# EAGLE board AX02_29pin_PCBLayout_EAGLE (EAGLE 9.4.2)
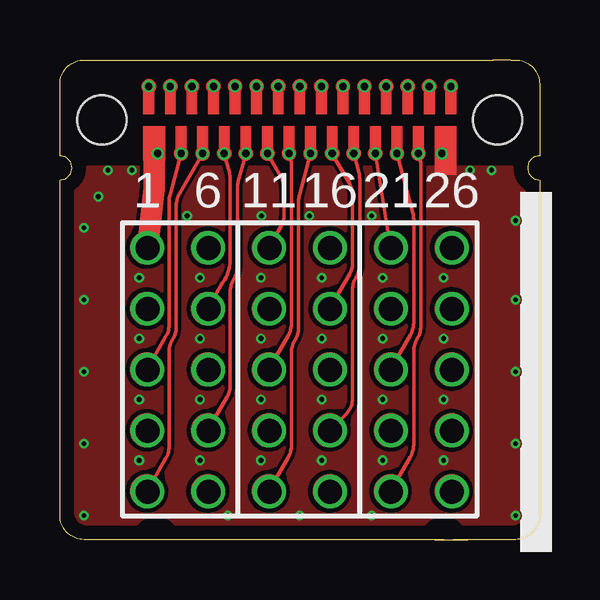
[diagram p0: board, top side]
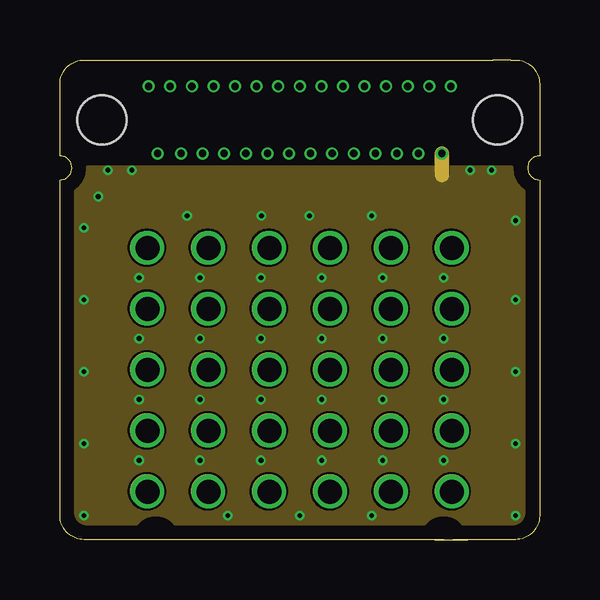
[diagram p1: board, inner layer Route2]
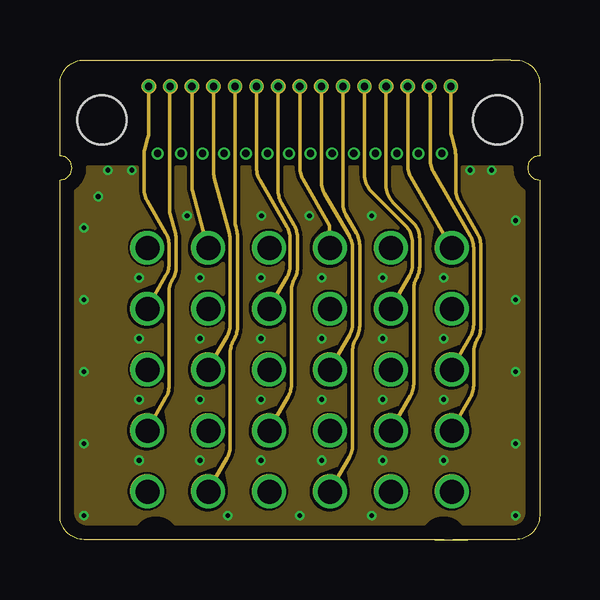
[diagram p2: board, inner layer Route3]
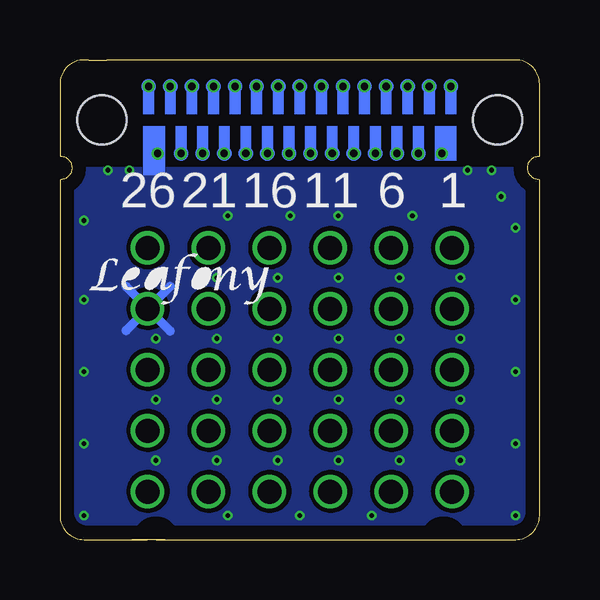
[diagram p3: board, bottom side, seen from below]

Size 20 x 20 mm. Coordinates in mm from the lower left corner, seen from the top.
Outline: 6,20 1,20 arc90 0,19 0,16 arc-180 0,15 0,1 arc90 1,0 16,0
Outline: 5.7,20 16,20
Outline: 15.05,20 18.05,20 18.8,20 19,20 arc-90 20,19 20,16 arc180 20,15 20,1 arc-90 19,0 16.38,0
Outline: 15.62,0 17,0
Copper layers (1*2+3*16): Top 0.035mm / dielectric 0.15mm / Route2 0.035mm / dielectric 0.15mm / Route3 0.035mm / dielectric 0.2mm / Bottom 0.035mm
Design rules "default *": minimum track width 0.01mm, minimum drill 0.01mm, track to track 0.01mm, track to pad 0.01mm, pad to pad 0.01mm, via to via 0.01mm, smd to smd 0.01mm, copper to edge 0.01mm, drill to drill 0.01mm, minimum pad ring 0.1mm, minimum via ring 0.1mm, stop-mask expansion 4mil, vias tented up to drill 0mil, thermal gap 10mil
Net classes: 0 default: width 0.15 mm, drill 0.3 mm; 1 power: width 0.15 mm, drill 0.3 mm

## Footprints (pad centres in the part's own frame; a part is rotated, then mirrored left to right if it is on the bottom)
29PAD = drill 0.3 pad 0.3: 3.3V -5.925,-1.4; A0 -4.5,1.4; A1 -3.6,1.4; A2 -2.7,1.4; A3 -1.8,1.4; A4 -0.9,1.4; A5 0,1.4; AREF -5.4,1.4; D0 0.9,1.4; D1 1.8,1.4; D2 2.7,1.4; D3 3.6,1.4; D4 4.5,1.4; D5 5.4,1.4; D6 -3.15,-1.4; D7 -2.25,-1.4; D8 -1.35,-1.4; D9 -0.45,-1.4; D10 0.45,-1.4; D11 1.35,-1.4; D12 2.25,-1.4; D13 3.15,-1.4; GRD 5.925,-1.4; RESET -4.05,-1.4; SDA 4.05,-1.4; SDL 4.95,-1.4; SWCLK 6.3,1.4; SWDIO -6.3,1.4; VBUS -4.95,-1.4 | hole 2.05: -8.25,0; 8.25,0
30PAD = drill 1 pad 1.4: 3.3V -6.35,12.16; 30PAD 6.35,2; A0 -3.81,12.16; A1 -3.81,7.08; A2 -3.81,2; A3 -1.27,9.62; A4 -1.27,4.54; A5 1.27,12.16; AREF -6.35,4.54; D0 1.27,7.08; D1 1.27,2; D2 3.81,9.62; D3 3.81,4.54; D4 6.35,12.16; D5 6.35,7.08; D6 -3.81,9.62; D7 -3.81,4.54; D8 -1.27,12.16; D9 -1.27,7.08; D10 -1.27,2; D11 1.27,9.62; D12 1.27,4.54; D13 3.81,12.16; GRD 6.35,9.62; REST -6.35,2; SDA 3.81,7.08; SDL 3.81,2; SWCLK 6.35,4.54; SWDIO -6.35,9.62; VBUS -6.35,7.08

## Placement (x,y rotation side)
E$1  [29PAD]  10,17.5 0 top
E$2  [30PAD]  10,0 0 top

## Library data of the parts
E$1 E$2 = 29PAD

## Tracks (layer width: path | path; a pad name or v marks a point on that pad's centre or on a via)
3.3V
  Top 0.9: 3.65,12.16 3.92,14.64 arc7 3.92,14.76 3.92,16.52
A0
  Route3 0.15: 6.17,12.17 5.53,14.53 arc-15 5.5,14.79 5.5,18.9
A1
  Route3 0.15: 6.4,18.9 6.4,15.36 arc15 6.43,15.1 7.07,12.74 arc-15 7.1,12.48 7.1,8.98 arc-30 6.97,8.48 6.17,7.09
A2
  Route3 0.15: 7.3,18.9 7.3,13.28 arc15 7.33,13.02 7.37,12.9 arc-15 7.4,12.64 7.4,8.85 arc-30 7.27,8.35 7.23,8.29 arc30 7.1,7.79 7.1,3.9 arc-30 6.97,3.4 6.17,2.01
A3
  Route3 0.15: 8.71,9.63 9.47,10.95 arc30 9.6,11.45 9.6,12.53 arc30 9.47,13.03 8.33,14.99 arc-30 8.2,15.49 8.2,18.9
A4
  Route3 0.15: 9.1,18.9 9.1,14.54 arc30 9.23,14.04 9.77,13.12 arc-30 9.9,12.62 9.9,11.32 arc-30 9.78,10.86 | 9.78,10.86 | 9.78,10.86 arc30 9.65,10.39 9.65,6.46 arc-30 9.52,5.96 8.71,4.55
A5
  Route3 0.15: 11.25,12.17 11.25,13.1 10.13,15.03 arc-30 10,15.53 10,18.9
AREF
  Route3 0.15: 3.63,4.55 4.42,5.92 arc30 4.55,6.42 4.55,10.32 arc-30 4.68,10.82 4.72,10.88 arc30 4.85,11.38 4.85,12.49 arc15 4.82,12.75 4.6,13.57 arc-15 4.56,13.83 4.56,18.49 arc-5 4.56,18.51 4.6,18.9
D0
  Route3 0.15: 11.25,7.09 12.07,8.51 arc30 12.2,9.01 12.2,12.15 arc30 12.07,12.65 11.03,14.44 arc-30 10.9,14.94 10.9,18.9
D1
  Route3 0.15: 11.25,2.01 12.07,3.43 arc30 12.2,3.93 12.2,7.86 arc-30 12.33,8.36 12.37,8.41 arc30 12.5,8.91 12.5,12.28 arc30 12.37,12.78 11.93,13.52 arc-30 11.8,14.02 11.8,18.9
D2
  Route3 0.15: 13.79,9.63 14.57,10.98 arc30 14.7,11.48 14.7,12.39 arc45 14.41,13.09 12.99,14.51 arc-45 12.7,15.21 12.7,18.9
D3
  Route3 0.15: 13.79,4.55 14.62,5.99 arc30 14.75,6.49 14.75,10.45 arc-30 14.88,10.92 | 14.88,10.92 | 14.88,10.92 arc30 15,11.38 15,12.54 arc45 14.71,13.24 13.89,14.06 arc-45 13.6,14.76 13.6,18.9
D4
  Route3 0.15: 14.5,18.9 14.5,15.6 arc30 14.63,15.1 16.33,12.17
D5
  Route3 0.15: 16.33,7.09 17.12,8.46 arc30 17.25,8.96 17.25,12.17 arc30 17.12,12.67 15.57,15.34 arc-30 15.44,15.84 15.44,18.49 arc5 15.44,18.51 15.4,18.9
D6
  Top 0.15: 6.85,16.1 7.07,15.29 arc-15 7.1,15.04 7.1,11.52 arc-30 6.79,10.72 6.17,9.63
D7
  Top 0.15: 7.75,16.1 7.43,14.92 arc15 7.4,14.66 7.4,11.39 arc-30 7.27,10.89 7.23,10.84 arc30 7.1,10.34 7.1,6.44 arc-30 6.97,5.94 6.17,4.55
D8
  Top 0.15: 8.71,12.17 9.22,13.05 arc30 9.35,13.55 9.35,14.62 arc30 9.22,15.12 8.65,16.1
D9
  Top 0.15: 8.71,7.09 9.52,8.49 arc30 9.65,8.99 9.65,15.73 9.55,16.1
D10
  Top 0.15: 10.45,16.1 9.98,14.36 arc15 9.95,14.1 9.95,8.84 arc-30 9.82,8.34 9.78,8.29 arc30 9.65,7.79 9.65,3.92 arc-30 9.52,3.42 8.71,2.01
D11
  Top 0.15: 11.35,16.1 12.07,14.86 arc-30 12.2,14.36 12.2,11.55 arc-30 12.07,11.05 11.25,9.63
D12
  Top 0.15: 12.25,16.1 12.47,15.29 arc-15 12.5,15.04 12.5,11.46 arc-30 12.37,10.96 12.33,10.91 arc30 12.2,10.41 12.2,5.88 arc-45 11.94,5.24 11.25,4.55
D13
  Top 0.15: 13.15,16.1 13.79,12.17
GND  (via drill 0.2 pad 0.4)
  Bottom 0.4: 16.33,9.63 15.4,8.71 | 16.33,9.63 17.25,8.71 | 16.33,9.63 15.41,10.55 | 16.33,9.63 17.24,10.55
  other vias: 10.4,13.5 13,13.5 8.4,13.5 5.3,13.5 3.3,10.92 5.84,10.92 8.38,10.92 10.92,10.92 13.46,10.92 16,10.92 3.3,8.38 5.84,8.38 8.38,8.38 10.92,8.38 13.46,8.38 16,8.38 3.3,5.84 5.84,5.84 8.38,5.84 10.92,5.84 13.46,5.84 16,5.84 3.3,3.3 5.84,3.3 8.38,3.3 10.92,3.3 13.46,3.3 16,3.3 18,15.4 3,15.4 2,15.4 19,13.3 1.6,14.3 1,13 1,10 1,7 13,1 10,1 7,1 1,4 1,1 19,10 19,7 19,4 19,1 17.1,15.4
  pour Top: 217 corners
  cutout Top: 16.33,11.27 arc-180 16.33,13.07 arc-180
  cutout Top: 16.33,8.73 arc-180 16.33,10.53 arc-180
  cutout Top: 16.33,6.19 arc-180 16.33,7.99 arc-180
  cutout Top: 16.33,3.65 arc-180 16.33,5.45 arc-180
  cutout Top: 16.33,1.11 arc-180 16.33,2.91 arc-180
  cutout Top: 11.25,1.11 arc-180 11.25,2.91 arc-180
  cutout Top: 6.17,1.11 arc-180 6.17,2.91 arc-180
  pour Top: 0.68,14.1 arc-90 0.6,14.18 0.6,14.54 arc-45 0.62,14.59 arc-10 0.63,14.6 arc55 1.1,15.5 1.1,15.53 arc-90 1.18,15.6 3.25,15.6 arc-90 3.33,15.53 3.33,14.76 arc-7 3.32,14.71 arc0 3.32,14.71 3.26,14.17 arc0 3.26,14.17 arc-1 3.26,14.17 3.26,14.17 arc-83 3.18,14.1
  pour Top: 5.22,14.1 arc-103 5.15,14.19 arc-17 5.23,14.4 5.89,15.55 arc-32 5.92,15.58 5.95,15.59 arc-28 5.98,15.6 6.69,15.6 arc-75 6.77,15.54 6.85,15.24 arc-15 6.88,15.04 6.88,14.18 arc-90 6.8,14.1
  pour Top: 7.7,14.1 arc-90 7.62,14.18 7.62,14.66 arc-15 7.65,14.86 7.83,15.54 arc-75 7.91,15.6 8.62,15.6 arc-28 8.65,15.59 8.68,15.58 arc-32 8.71,15.55 9.02,15.01 arc-30 9.12,14.62 9.12,14.18 arc-90 9.05,14.1
  pour Top: 10.25,14.1 arc-96 10.18,14.18 arc-9 10.2,14.3 10.53,15.54 arc-75 10.61,15.6 11.32,15.6 arc-28 11.35,15.59 11.38,15.58 arc-32 11.41,15.55 11.87,14.75 arc-30 11.97,14.36 11.97,14.18 arc-90 11.9,14.1
  pour Top: 12.8,14.1 arc-90 12.72,14.18 12.72,15.04 arc15 12.68,15.35 arc0 12.68,15.35 12.64,15.51 arc-105 12.71,15.6 12.94,15.6 arc-81 13.01,15.54 13.23,14.19 arc-99 13.16,14.1
  pour Top: 15.35,14.1 arc-90 15.28,14.18 15.28,15.53 arc-90 15.35,15.6 18.82,15.6 arc-90 18.9,15.53 18.9,15.5 arc55 19.37,14.6 arc-55 19.4,14.54 19.4,14.18 arc-90 19.32,14.1
  pour Route2: 1.1,0.6 arc-90 0.6,1.1 0.6,14.54 arc-45 0.62,14.59 arc-10 0.63,14.6 arc55 1.1,15.5 1.1,15.53 arc-90 1.18,15.6 18.82,15.6 arc-90 18.9,15.53 18.9,15.5 arc55 19.37,14.6 arc-55 19.4,14.54 19.4,1.1 arc-90 18.9,0.6 16.8,0.6 arc-45 16.75,0.62 arc-5 16.75,0.63 arc0 16.75,0.63 arc100 15.25,0.63 arc-50 15.2,0.6 4.8,0.6 arc-45 4.75,0.62 arc-5 4.75,0.63 arc0 4.75,0.63 arc100 3.25,0.63 arc-50 3.2,0.6
  cutout Route2: 3.63,8.83 arc-180 3.63,10.43 arc-180
  cutout Route2: 3.63,11.37 arc-180 3.63,12.97 arc-180
  cutout Route2: 6.17,11.37 arc-180 6.17,12.97 arc-180
  cutout Route2: 6.17,8.83 arc-180 6.17,10.43 arc-180
  cutout Route2: 8.71,8.83 arc-180 8.71,10.43 arc-180
  cutout Route2: 8.71,11.37 arc-180 8.71,12.97 arc-180
  cutout Route2: 11.25,11.37 arc-180 11.25,12.97 arc-180
  cutout Route2: 11.25,8.83 arc-180 11.25,10.43 arc-180
  cutout Route2: 13.79,8.83 arc-180 13.79,10.43 arc-180
  cutout Route2: 13.79,11.37 arc-180 13.79,12.97 arc-180
  cutout Route2: 16.33,11.37 arc-180 16.33,12.97 arc-180
  cutout Route2: 16.33,8.83 arc-180 16.33,10.43 arc-180
  cutout Route2: 3.63,6.29 arc-180 3.63,7.89 arc-180
  cutout Route2: 6.17,6.29 arc-180 6.17,7.89 arc-180
  cutout Route2: 8.71,6.29 arc-180 8.71,7.89 arc-180
  cutout Route2: 11.25,6.29 arc-180 11.25,7.89 arc-180
  cutout Route2: 13.79,6.29 arc-180 13.79,7.89 arc-180
  cutout Route2: 16.33,6.29 arc-180 16.33,7.89 arc-180
  cutout Route2: 16.33,3.75 arc-180 16.33,5.35 arc-180
  cutout Route2: 13.79,3.75 arc-180 13.79,5.35 arc-180
  cutout Route2: 11.25,3.75 arc-180 11.25,5.35 arc-180
  cutout Route2: 8.71,3.75 arc-180 8.71,5.35 arc-180
  cutout Route2: 6.17,3.75 arc-180 6.17,5.35 arc-180
  cutout Route2: 3.63,3.75 arc-180 3.63,5.35 arc-180
  cutout Route2: 3.63,1.21 arc-180 3.63,2.81 arc-180
  cutout Route2: 6.17,1.21 arc-180 6.17,2.81 arc-180
  cutout Route2: 8.71,1.21 arc-180 8.71,2.81 arc-180
  cutout Route2: 11.25,1.21 arc-180 11.25,2.81 arc-180
  cutout Route2: 13.79,1.21 arc-180 13.79,2.81 arc-180
  cutout Route2: 16.33,1.21 arc-180 16.33,2.81 arc-180
  pour Route3: 313 corners
  cutout Route3: 16.33,1.21 arc-180 16.33,2.81 arc-180
  cutout Route3: 13.79,1.21 arc-180 13.79,2.81 arc-180
  cutout Route3: 8.71,1.21 arc-180 8.71,2.81 arc-180
  cutout Route3: 3.63,1.21 arc-180 3.63,2.81 arc-180
  pour Bottom: 1.1,0.6 arc-90 0.6,1.1 0.6,14.43 arc-90 0.68,14.5 19.32,14.5 arc-90 19.4,14.43 19.4,1.1 arc-90 18.9,0.6 16.8,0.6 arc-45 16.75,0.62 arc-5 16.75,0.63 arc0 16.75,0.63 arc100 15.25,0.63 arc-23 15.23,0.61 15.23,0.61 arc-27 15.2,0.6 4.8,0.6 arc-45 4.75,0.62 arc-5 4.75,0.63 arc0 4.75,0.63 arc100 3.25,0.63 arc-23 3.23,0.61 3.23,0.61 arc-27 3.2,0.6
  cutout Bottom: 16.33,11.27 arc-180 16.33,13.07 arc-180
  cutout Bottom: 13.79,11.27 arc-180 13.79,13.07 arc-180
  cutout Bottom: 11.25,11.27 arc-180 11.25,13.07 arc-180
  cutout Bottom: 8.71,11.27 arc-180 8.71,13.07 arc-180
  cutout Bottom: 6.17,11.27 arc-180 6.17,13.07 arc-180
  cutout Bottom: 3.63,11.27 arc-180 3.63,13.07 arc-180
  cutout Bottom: 3.63,8.73 arc-180 3.63,10.53 arc-180
  cutout Bottom: 6.17,8.73 arc-180 6.17,10.53 arc-180
  cutout Bottom: 8.71,8.73 arc-180 8.71,10.53 arc-180
  cutout Bottom: 11.25,8.73 arc-180 11.25,10.53 arc-180
  cutout Bottom: 13.79,8.73 arc-180 13.79,10.53 arc-180
  cutout Bottom: 16.33,8.73 arc-180 16.33,10.53 arc-180
  cutout Bottom: 16.33,6.19 arc-180 16.33,7.99 arc-180
  cutout Bottom: 13.79,6.19 arc-180 13.79,7.99 arc-180
  cutout Bottom: 11.25,6.19 arc-180 11.25,7.99 arc-180
  cutout Bottom: 8.71,6.19 arc-180 8.71,7.99 arc-180
  cutout Bottom: 6.17,6.19 arc-180 6.17,7.99 arc-180
  cutout Bottom: 3.63,6.19 arc-180 3.63,7.99 arc-180
  cutout Bottom: 3.63,3.65 arc-180 3.63,5.45 arc-180
  cutout Bottom: 6.17,3.65 arc-180 6.17,5.45 arc-180
  cutout Bottom: 8.71,3.65 arc-180 8.71,5.45 arc-180
  cutout Bottom: 11.25,3.65 arc-180 11.25,5.45 arc-180
  cutout Bottom: 13.79,3.65 arc-180 13.79,5.45 arc-180
  cutout Bottom: 16.33,3.65 arc-180 16.33,5.45 arc-180
  cutout Bottom: 16.33,1.11 arc-180 16.33,2.91 arc-180
  cutout Bottom: 13.79,1.11 arc-180 13.79,2.91 arc-180
  cutout Bottom: 11.25,1.11 arc-180 11.25,2.91 arc-180
  cutout Bottom: 8.71,1.11 arc-180 8.71,2.91 arc-180
  cutout Bottom: 6.17,1.11 arc-180 6.17,2.91 arc-180
  cutout Bottom: 3.63,1.11 arc-180 3.63,2.91 arc-180
  pour Bottom: 0.68,14.1 arc-90 0.6,14.18 0.6,14.54 arc-45 0.62,14.59 arc-10 0.63,14.6 arc55 1.1,15.5 1.1,15.53 18.9,15.53 18.9,15.5 arc55 19.37,14.6 arc-28 19.39,14.57 arc-27 19.4,14.54 19.4,14.18 arc-90 19.32,14.1
RESET
  Top 0.15: 5.95,16.1 4.98,14.43 arc30 4.85,13.93 4.85,8.88 arc-30 4.72,8.38 4.68,8.32 arc30 4.55,7.82 4.55,3.88 arc-30 4.42,3.38 3.63,2.01
S$1
  Top 0.15: 5.05,16.1 4.58,14.36 arc15 4.55,14.1 4.55,8.96 arc-30 4.42,8.46 3.63,7.09
S$3
  Route2 0.6: 15.93,16.1 15.93,15.2
SCL
  Top 0.15: 13.79,2.01 14.62,3.45 arc30 14.75,3.95 14.75,7.85 arc-30 14.88,8.35 14.92,8.4 arc30 15.05,8.9 15.05,15.73 14.95,16.1
SDA
  Top 0.15: 13.79,7.09 14.62,8.53 arc30 14.75,9.03 14.75,13.36 arc15 14.72,13.62 14.05,16.1
SWCLK
  Route3 0.15: 16.33,4.55 17.12,5.92 arc30 17.25,6.42 17.25,7.81 arc-30 17.38,8.31 17.42,8.36 arc30 17.55,8.86 17.55,12.25 arc30 17.42,12.75 16.63,14.11 arc-30 16.5,14.61 16.5,16.05 arc15 16.47,16.3 16.33,16.8 arc-15 16.3,17.05 16.3,18.9
SWDIO
  Route3 0.15: 3.7,18.9 3.7,17 arc-15 3.67,16.75 3.53,16.25 arc15 3.5,15.99 3.5,14.63 arc30 3.63,14.13 4.42,12.78 arc-30 4.55,12.28 4.55,11.5 arc-30 4.42,11 3.63,9.63
(copper drawn outside any net)
  shapes: Bottom area x1, Route2 circle x32, Route3 circle x50, Top area x1, Top circle x32

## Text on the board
tPlace: 1 | 6 | 11 | 16 | 21 | 26
bPlace: 1 | 6 | 11 | 16 | 21 | 26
